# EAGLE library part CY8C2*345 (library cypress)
PSoC® Programmable System-on-Chip TM M8C Processor Speeds up to 24 MHz Source: http://www.cypress.com .. CY8C213452.pdf
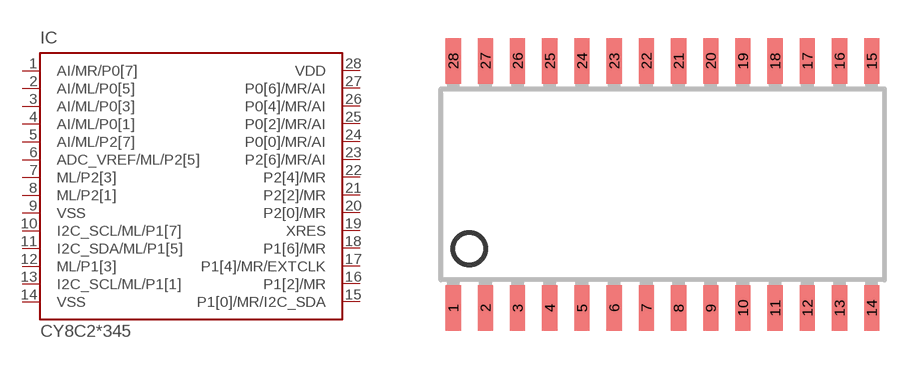
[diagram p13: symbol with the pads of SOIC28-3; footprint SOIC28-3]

Designator prefix IC

## CY8C21345 (OC_FARNELL: unknown; OC_NEWARK: unknown), CY8C22345 (MPN: CY3250-22345; OC_FARNELL: unknown; OC_NEWARK: 50R9266)  [SOIC28-3]
1  AI/MR/P0[7]
2  AI/ML/P0[5]
3  AI/ML/P0[3]
4  AI/ML/P0[1]
5  AI/ML/P2[7]
6  ADC_VREF/ML/P2[5]
7  ML/P2[3]
8  ML/P2[1]
9  VSS  pwr
10  I2C_SCL/ML/P1[7]
11  I2C_SDA/ML/P1[5]
12  ML/P1[3]
13  I2C_SCL/ML/P1[1]
14  VSS  pwr
15  P1[0]/MR/I2C_SDA
16  P1[2]/MR
17  P1[4]/MR/EXTCLK
18  P1[6]/MR
19  XRES  in
20  P2[0]/MR
21  P2[2]/MR
22  P2[4]/MR
23  P2[6]/MR/AI
24  P0[0]/MR/AI
25  P0[2]/MR/AI
26  P0[4]/MR/AI
27  P0[6]/MR/AI
28  VDD  pwr

## Footprint SOIC28-3 (pad centres in mm)
28-Pin SOIC Body 7.63 mm Source: http://www.cypress.com .. CY8C21345.pdf
smd 0.6 x 1.8: 1 -8.255,-4.87; 2 -6.985,-4.87; 3 -5.715,-4.87; 4 -4.445,-4.87; 5 -3.175,-4.87; 6 -1.905,-4.87; 7 -0.635,-4.87; 8 0.635,-4.87; 9 1.905,-4.87; 10 3.175,-4.87; 11 4.445,-4.87; 12 5.715,-4.87; 13 6.985,-4.87; 14 8.255,-4.87; 15 8.255,4.87; 16 6.985,4.87; 17 5.715,4.87; 18 4.445,4.87; 19 3.175,4.87; 20 1.905,4.87; 21 0.635,4.87; 22 -0.635,4.87; 23 -1.905,4.87; 24 -3.175,4.87; 25 -4.445,4.87; 26 -5.715,4.87; 27 -6.985,4.87; 28 -8.255,4.87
